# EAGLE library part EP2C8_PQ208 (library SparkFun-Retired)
Altera Cyclone2 FPGA, PQFP-208 Not in catalog
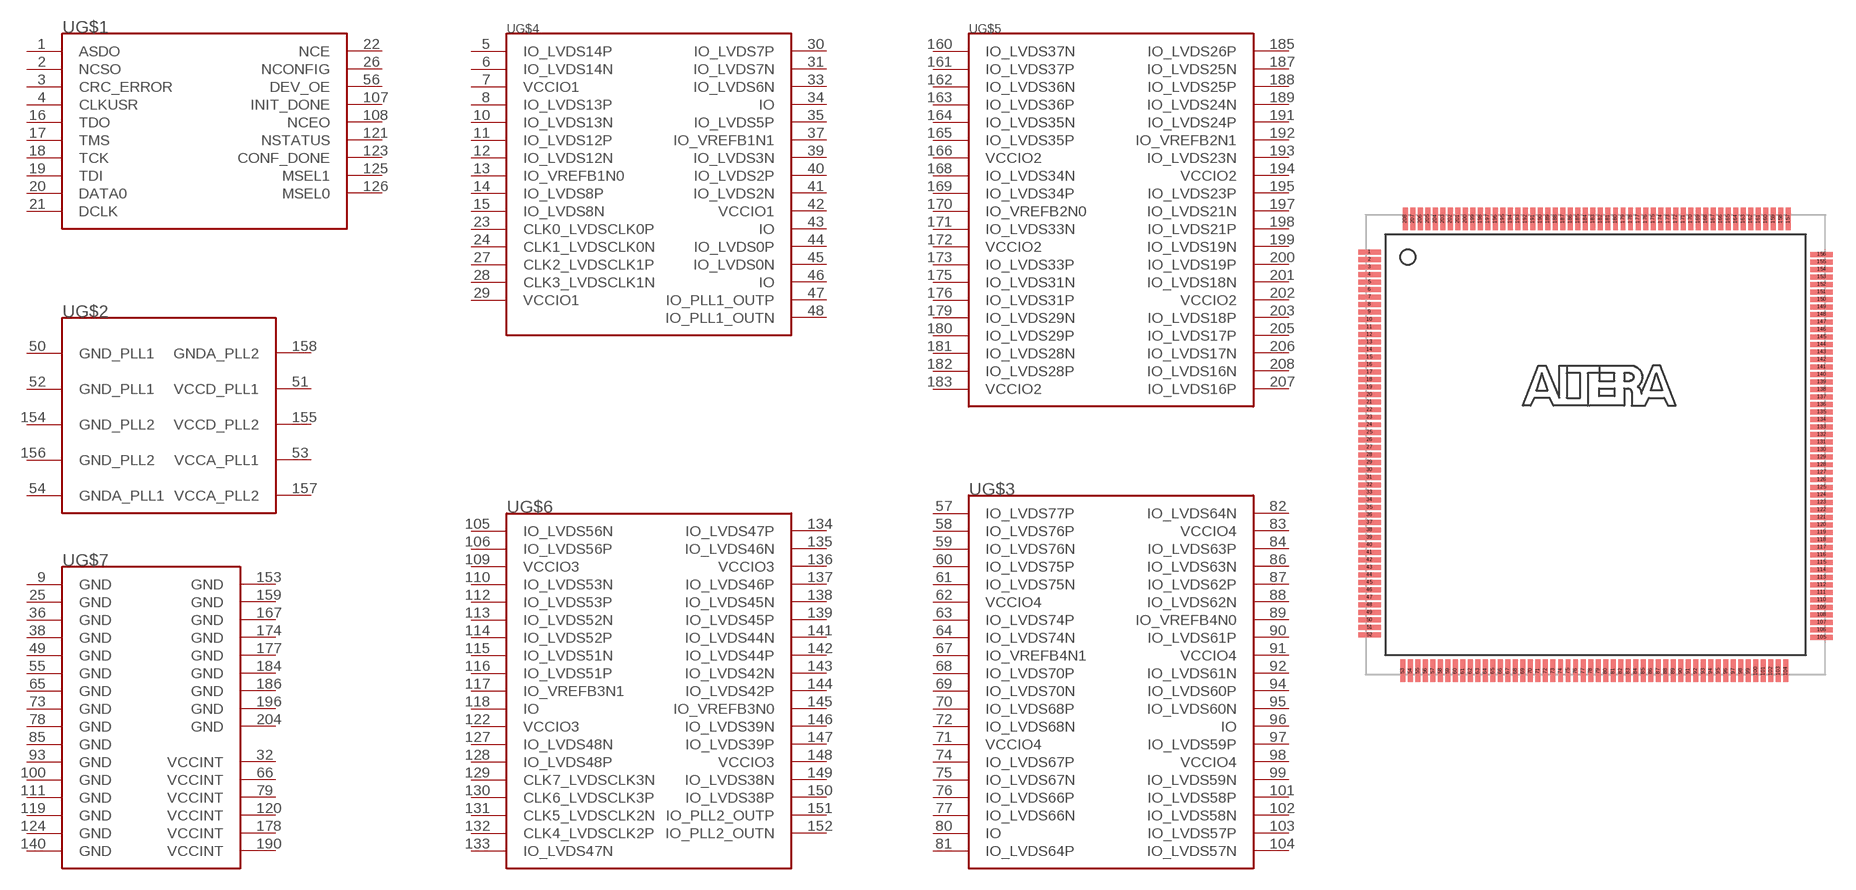
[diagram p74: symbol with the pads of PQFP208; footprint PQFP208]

Designator prefix -; gates G$2=EP2C20_PQ208_PLL G$6=EP2C20_PQ208_B3 G$4=EP2C20_PQ208_B1 G$3=EP2C20_PQ208_B4 G$7=EP2C20_PQ208_POWER G$5=EP2C20_PQ208_B2 G$1=EP2C20_PQ208_CONFIG

## EP2C8_PQ208  [PQFP208]
1  G$1:ASDO
2  G$1:NCSO
3  G$1:CRC_ERROR
4  G$1:CLKUSR
5  G$4:IO_LVDS14P
6  G$4:IO_LVDS14N
7  G$4:VCCIO1
8  G$4:IO_LVDS13P
9  G$7:GND  pwr
10  G$4:IO_LVDS13N
11  G$4:IO_LVDS12P
12  G$4:IO_LVDS12N
13  G$4:IO_VREFB1N0
14  G$4:IO_LVDS8P
15  G$4:IO_LVDS8N
16  G$1:TDO
17  G$1:TMS
18  G$1:TCK
19  G$1:TDI
20  G$1:DATA0
21  G$1:DCLK
22  G$1:NCE
23  G$4:CLK0_LVDSCLK0P
24  G$4:CLK1_LVDSCLK0N
25  G$7:GND  pwr
26  G$1:NCONFIG
27  G$4:CLK2_LVDSCLK1P
28  G$4:CLK3_LVDSCLK1N
29  G$4:VCCIO1
30  G$4:IO_LVDS7P
31  G$4:IO_LVDS7N
32  G$7:VCCINT  pwr
33  G$4:IO_LVDS6N
34  G$4:IO
35  G$4:IO_LVDS5P
36  G$7:GND  pwr
37  G$4:IO_VREFB1N1
38  G$7:GND  pwr
39  G$4:IO_LVDS3N
40  G$4:IO_LVDS2P
41  G$4:IO_LVDS2N
42  G$4:VCCIO1
43  G$4:IO
44  G$4:IO_LVDS0P
45  G$4:IO_LVDS0N
46  G$4:IO
47  G$4:IO_PLL1_OUTP
48  G$4:IO_PLL1_OUTN
49  G$7:GND  pwr
50  G$2:GND_PLL1  pwr
51  G$2:VCCD_PLL1  pwr
52  G$2:GND_PLL1  pwr
53  G$2:VCCA_PLL1  pwr
54  G$2:GNDA_PLL1  pwr
55  G$7:GND  pwr
56  G$1:DEV_OE
57  G$3:IO_LVDS77P
58  G$3:IO_LVDS76P
59  G$3:IO_LVDS76N
60  G$3:IO_LVDS75P
61  G$3:IO_LVDS75N
62  G$3:VCCIO4
63  G$3:IO_LVDS74P
64  G$3:IO_LVDS74N
65  G$7:GND  pwr
66  G$7:VCCINT  pwr
67  G$3:IO_VREFB4N1
68  G$3:IO_LVDS70P
69  G$3:IO_LVDS70N
70  G$3:IO_LVDS68P
71  G$3:VCCIO4
72  G$3:IO_LVDS68N
73  G$7:GND  pwr
74  G$3:IO_LVDS67P
75  G$3:IO_LVDS67N
76  G$3:IO_LVDS66P
77  G$3:IO_LVDS66N
78  G$7:GND  pwr
79  G$7:VCCINT  pwr
80  G$3:IO
81  G$3:IO_LVDS64P
82  G$3:IO_LVDS64N
83  G$3:VCCIO4
84  G$3:IO_LVDS63P
85  G$7:GND  pwr
86  G$3:IO_LVDS63N
87  G$3:IO_LVDS62P
88  G$3:IO_LVDS62N
89  G$3:IO_VREFB4N0
90  G$3:IO_LVDS61P
91  G$3:VCCIO4
92  G$3:IO_LVDS61N
93  G$7:GND  pwr
94  G$3:IO_LVDS60P
95  G$3:IO_LVDS60N
96  G$3:IO
97  G$3:IO_LVDS59P
98  G$3:VCCIO4
99  G$3:IO_LVDS59N
100  G$7:GND  pwr
101  G$3:IO_LVDS58P
102  G$3:IO_LVDS58N
103  G$3:IO_LVDS57P
104  G$3:IO_LVDS57N
105  G$6:IO_LVDS56N
106  G$6:IO_LVDS56P
107  G$1:INIT_DONE
108  G$1:NCEO
109  G$6:VCCIO3
110  G$6:IO_LVDS53N
111  G$7:GND  pwr
112  G$6:IO_LVDS53P
113  G$6:IO_LVDS52N
114  G$6:IO_LVDS52P
115  G$6:IO_LVDS51N
116  G$6:IO_LVDS51P
117  G$6:IO_VREFB3N1
118  G$6:IO
119  G$7:GND  pwr
120  G$7:VCCINT  pwr
121  G$1:NSTATUS
122  G$6:VCCIO3
123  G$1:CONF_DONE
124  G$7:GND
125  G$1:MSEL1
126  G$1:MSEL0
127  G$6:IO_LVDS48N
128  G$6:IO_LVDS48P
129  G$6:CLK7_LVDSCLK3N
130  G$6:CLK6_LVDSCLK3P
131  G$6:CLK5_LVDSCLK2N
132  G$6:CLK4_LVDSCLK2P
133  G$6:IO_LVDS47N
134  G$6:IO_LVDS47P
135  G$6:IO_LVDS46N
136  G$6:VCCIO3
137  G$6:IO_LVDS46P
138  G$6:IO_LVDS45N
139  G$6:IO_LVDS45P
140  G$7:GND
141  G$6:IO_LVDS44N
142  G$6:IO_LVDS44P
143  G$6:IO_LVDS42N
144  G$6:IO_LVDS42P
145  G$6:IO_VREFB3N0
146  G$6:IO_LVDS39N
147  G$6:IO_LVDS39P
148  G$6:VCCIO3
149  G$6:IO_LVDS38N
150  G$6:IO_LVDS38P
151  G$6:IO_PLL2_OUTP
152  G$6:IO_PLL2_OUTN
153  G$7:GND
154  G$2:GND_PLL2  pwr
155  G$2:VCCD_PLL2  pwr
156  G$2:GND_PLL2  pwr
157  G$2:VCCA_PLL2  pwr
158  G$2:GNDA_PLL2  pwr
159  G$7:GND
160  G$5:IO_LVDS37N
161  G$5:IO_LVDS37P
162  G$5:IO_LVDS36N
163  G$5:IO_LVDS36P
164  G$5:IO_LVDS35N
165  G$5:IO_LVDS35P
166  G$5:VCCIO2
167  G$7:GND
168  G$5:IO_LVDS34N
169  G$5:IO_LVDS34P
170  G$5:IO_VREFB2N0
171  G$5:IO_LVDS33N
172  G$5:VCCIO2
173  G$5:IO_LVDS33P
174  G$7:GND
175  G$5:IO_LVDS31N
176  G$5:IO_LVDS31P
177  G$7:GND
178  G$7:VCCINT  pwr
179  G$5:IO_LVDS29N
180  G$5:IO_LVDS29P
181  G$5:IO_LVDS28N
182  G$5:IO_LVDS28P
183  G$5:VCCIO2
184  G$7:GND
185  G$5:IO_LVDS26P
186  G$7:GND
187  G$5:IO_LVDS25N
188  G$5:IO_LVDS25P
189  G$5:IO_LVDS24N
190  G$7:VCCINT  pwr
191  G$5:IO_LVDS24P
192  G$5:IO_VREFB2N1
193  G$5:IO_LVDS23N
194  G$5:VCCIO2
195  G$5:IO_LVDS23P
196  G$7:GND
197  G$5:IO_LVDS21N
198  G$5:IO_LVDS21P
199  G$5:IO_LVDS19N
200  G$5:IO_LVDS19P
201  G$5:IO_LVDS18N
202  G$5:VCCIO2
203  G$5:IO_LVDS18P
204  G$7:GND
205  G$5:IO_LVDS17P
206  G$5:IO_LVDS17N
207  G$5:IO_LVDS16P
208  G$5:IO_LVDS16N

## Footprint PQFP208 (pad centres in mm)
smd 1.5 x 0.33: 1 -15.05,12.83; 2 -15.05,12.33; 3 -15.05,11.83; 4 -15.05,11.33; 5 -15.05,10.83; 6 -15.05,10.33; 7 -15.05,9.83; 8 -15.05,9.33; 9 -15.05,8.83; 10 -15.05,8.33; 11 -15.05,7.83; 12 -15.05,7.33; 13 -15.05,6.83; 14 -15.05,6.33; 15 -15.05,5.83; 16 -15.05,5.33; 17 -15.05,4.83; 18 -15.05,4.33; 19 -15.05,3.83; 20 -15.05,3.33; 21 -15.05,2.83; 22 -15.05,2.33; 23 -15.05,1.83; 24 -15.05,1.33; 25 -15.05,0.83; 26 -15.05,0.33; 27 -15.05,-0.17; 28 -15.05,-0.67; 29 -15.05,-1.17; 30 -15.05,-1.67; 31 -15.05,-2.17; 32 -15.05,-2.67; 33 -15.05,-3.17; 34 -15.05,-3.67; 35 -15.05,-4.17; 36 -15.05,-4.67; 37 -15.05,-5.17; 38 -15.05,-5.67; 39 -15.05,-6.17; 40 -15.05,-6.67; 41 -15.05,-7.17; 42 -15.05,-7.67; 43 -15.05,-8.17; 44 -15.05,-8.67; 45 -15.05,-9.17; 46 -15.05,-9.67; 47 -15.05,-10.17; 48 -15.05,-10.67; 49 -15.05,-11.17; 50 -15.05,-11.67; 51 -15.04,-12.17; 52 -15.05,-12.67; 105 15.05,-12.83; 106 15.05,-12.33; 107 15.05,-11.83; 108 15.05,-11.33; 109 15.05,-10.83; 110 15.05,-10.33; 111 15.05,-9.83; 112 15.05,-9.33; 113 15.05,-8.83; 114 15.05,-8.33; 115 15.05,-7.83; 116 15.05,-7.33; 117 15.05,-6.83; 118 15.05,-6.33; 119 15.05,-5.83; 120 15.05,-5.33; 121 15.05,-4.83; 122 15.05,-4.33; 123 15.05,-3.83; 124 15.05,-3.33; 125 15.05,-2.83; 126 15.05,-2.33; 127 15.05,-1.83; 128 15.05,-1.33; 129 15.05,-0.83; 130 15.05,-0.33; 131 15.05,0.17; 132 15.05,0.67; 133 15.05,1.17; 134 15.05,1.67; 135 15.05,2.17; 136 15.05,2.67; 137 15.05,3.17; 138 15.05,3.67; 139 15.05,4.17; 140 15.05,4.67; 141 15.05,5.17; 142 15.05,5.67; 143 15.05,6.17; 144 15.05,6.67; 145 15.05,7.17; 146 15.05,7.67; 147 15.05,8.17; 148 15.05,8.67; 149 15.05,9.17; 150 15.05,9.67; 151 15.05,10.17; 152 15.05,10.67; 153 15.05,11.17; 154 15.05,11.67; 155 15.04,12.17; 156 15.05,12.67
smd 0.33 x 1.5: 53 -12.83,-15.05; 54 -12.33,-15.05; 55 -11.83,-15.05; 56 -11.33,-15.05; 57 -10.83,-15.05; 58 -10.33,-15.05; 59 -9.83,-15.05; 60 -9.33,-15.05; 61 -8.83,-15.05; 62 -8.33,-15.05; 63 -7.83,-15.05; 64 -7.33,-15.05; 65 -6.83,-15.05; 66 -6.33,-15.05; 67 -5.83,-15.05; 68 -5.33,-15.05; 69 -4.83,-15.05; 70 -4.33,-15.05; 71 -3.83,-15.05; 72 -3.33,-15.05; 73 -2.83,-15.05; 74 -2.33,-15.05; 75 -1.83,-15.05; 76 -1.33,-15.05; 77 -0.83,-15.05; 78 -0.33,-15.05; 79 0.17,-15.05; 80 0.67,-15.05; 81 1.17,-15.05; 82 1.67,-15.05; 83 2.17,-15.05; 84 2.67,-15.05; 85 3.17,-15.05; 86 3.67,-15.05; 87 4.17,-15.05; 88 4.67,-15.05; 89 5.17,-15.05; 90 5.67,-15.05; 91 6.17,-15.05; 92 6.67,-15.05; 93 7.17,-15.05; 94 7.67,-15.05; 95 8.17,-15.05; 96 8.67,-15.05; 97 9.17,-15.05; 98 9.67,-15.05; 99 10.17,-15.05; 100 10.67,-15.05; 101 11.17,-15.05; 102 11.67,-15.05; 103 12.17,-15.04; 104 12.67,-15.05; 157 12.83,15.05; 158 12.33,15.05; 159 11.83,15.05; 160 11.33,15.05; 161 10.83,15.05; 162 10.33,15.05; 163 9.83,15.05; 164 9.33,15.05; 165 8.83,15.05; 166 8.33,15.05; 167 7.83,15.05; 168 7.33,15.05; 169 6.83,15.05; 170 6.33,15.05; 171 5.83,15.05; 172 5.33,15.05; 173 4.83,15.05; 174 4.33,15.05; 175 3.83,15.05; 176 3.33,15.05; 177 2.83,15.05; 178 2.33,15.05; 179 1.83,15.05; 180 1.33,15.05; 181 0.83,15.05; 182 0.33,15.05; 183 -0.17,15.05; 184 -0.67,15.05; 185 -1.17,15.05; 186 -1.67,15.05; 187 -2.17,15.05; 188 -2.67,15.05; 189 -3.17,15.05; 190 -3.67,15.05; 191 -4.17,15.05; 192 -4.67,15.05; 193 -5.17,15.05; 194 -5.67,15.05; 195 -6.17,15.05; 196 -6.67,15.05; 197 -7.17,15.05; 198 -7.67,15.05; 199 -8.17,15.05; 200 -8.67,15.05; 201 -9.17,15.05; 202 -9.67,15.05; 203 -10.17,15.05; 204 -10.67,15.05; 205 -11.17,15.05; 206 -11.67,15.05; 207 -12.168,15.049; 208 -12.67,15.05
